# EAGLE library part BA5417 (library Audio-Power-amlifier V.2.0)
High-output dual power amplifier
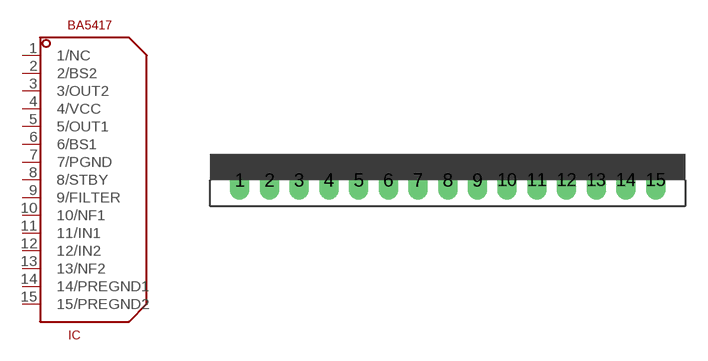
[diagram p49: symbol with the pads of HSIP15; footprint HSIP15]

Designator prefix IC

## BA5417  [HSIP15]
1  1/NC  nc
2  2/BS2
3  3/OUT2  out
4  4/VCC  pwr
5  5/OUT1  out
6  6/BS1
7  7/PGND  pwr
8  8/STBY
9  9/FILTER
10  10/NF1
11  11/IN1  in
12  12/IN2  in
13  13/NF2
14  14/PREGND1  pwr
15  15/PREGND2  pwr

## Footprint HSIP15 (pad centres in mm)
drill 0.8 long: 1 -13.97,-1.27; 2 -11.97,-1.27; 3 -9.97,-1.27; 4 -7.97,-1.27; 5 -5.97,-1.27; 6 -3.97,-1.27; 7 -1.97,-1.27; 8 0.03,-1.27; 9 2.03,-1.27; 10 4.03,-1.27; 11 6.03,-1.27; 12 8.03,-1.27; 13 10.03,-1.27; 14 12.03,-1.27; 15 14.03,-1.27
